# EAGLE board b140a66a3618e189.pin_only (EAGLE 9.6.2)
REV: B

Size 19.05 x 21.59 mm. Coordinates in mm from the lower left corner, seen from the top.
Outline: 19.05,19.05 19.05,2.54 arc-90 16.51,0 2.54,0 arc-90 0,2.54 0,19.05 arc-90 2.54,21.59 16.51,21.59 arc-90 19.05,19.05
Copper layers (1*16): Top 0.035mm / dielectric 1.5mm / Bottom 0.035mm
Design rules "adafruit *": minimum track width 8mil, minimum drill 15.5mil, track to track 8mil, track to pad 8mil, pad to pad 8mil, via to via 8mil, smd to smd 8mil, copper to edge 10mil, drill to drill 8mil, minimum pad ring 10mil, minimum via ring 8mil, stop-mask expansion 2mil, vias tented up to drill 20mil, thermal gap 10mil
Net classes: 1 highpower: width 0.305 mm, drill 0.483 mm; 2 lowpower: width 0.254 mm, drill 0.483 mm
Holes 2.54 mm at 17.14,16.51 1.91,5.08

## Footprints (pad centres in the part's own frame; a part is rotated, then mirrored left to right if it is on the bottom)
0603-NO = smd 1.075 x 1: 1 -0.85,0; 2 0.85,0
SOD-323 = smd 1.35 x 0.8: A 1.27,0; C -1.27,0
FIDUCIAL_1MM = smd 1 x 1: 1 0,0
1X05_ROUND_70 = drill 1 pad 1.778: 1 -5.08,0; 2 -2.54,0; 3 0,0; 4 2.54,0; 5 5.08,0
1X02_ROUND = drill 1 pad 1.778: 1 -1.27,0; 2 1.27,0
NEO3535_REVERSE = smd 1.2 x 0.9 bottom: 1-VDD 2.65,-0.75; 2-DOUT 2.65,0.75; 3-GND -2.65,0.75; 4-DIN -2.65,-0.75
KAILH_SOCKET = smd 2.55 x 2.5 bottom: 1 6.09,5.08; 2 -7.36,2.5 | hole 3.9: 0,0 | hole 3.063: 2.54,5.08; -3.81,2.54 | hole 1.813: 5.08,0; -5.08,0

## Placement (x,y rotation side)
C1  1uF  [0603-NO]  14.73,6.86 0 top
D1  1N4148  [SOD-323]  6.48,9.78 90 top
FID3  FIDUCIAL_1MM  [FIDUCIAL_1MM]  17.78,5.84 0 top
FID4  FIDUCIAL_1MM  [FIDUCIAL_1MM]  1.78,20.07 0 top
JP1  [1X05_ROUND_70]  9.53,19.68 0 bottom
JP2  [1X02_ROUND]  17.78,9.53 90 bottom
JP3  [1X05_ROUND_70]  9.53,1.91 0 bottom
JP4  [1X02_ROUND]  1.27,9.53 90 bottom
LED1  WS2812B_SK6812E  [NEO3535_REVERSE]  9.53,6.1 180 bottom
SW1  [KAILH_SOCKET]  9.53,10.79 0 bottom
U$1  [PCBFEAT-REV-040]  17.53,19.18 0 top
U$2  [ADAFRUIT_3.5MM]  15.24,0.76 0 top

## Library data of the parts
C1 D1 JP1-JP4 LED1 U$2 = microbuilder
FID3 FID4 = microbuilder; BOM: EXCLUDE
SW1 = adafruit_electromech
U$1 = microbuilder; REV: B

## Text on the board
tPlace: NeoKey | C | C | OUT | IN | S- | S+ | VDD | IN | G
bPlace: C | A | O | - | + | C | A | I | - | +

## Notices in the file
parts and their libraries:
microbuilder: This work is placed in the public domain, and may be freely used for commercial and non-commercial work with the following conditions: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
